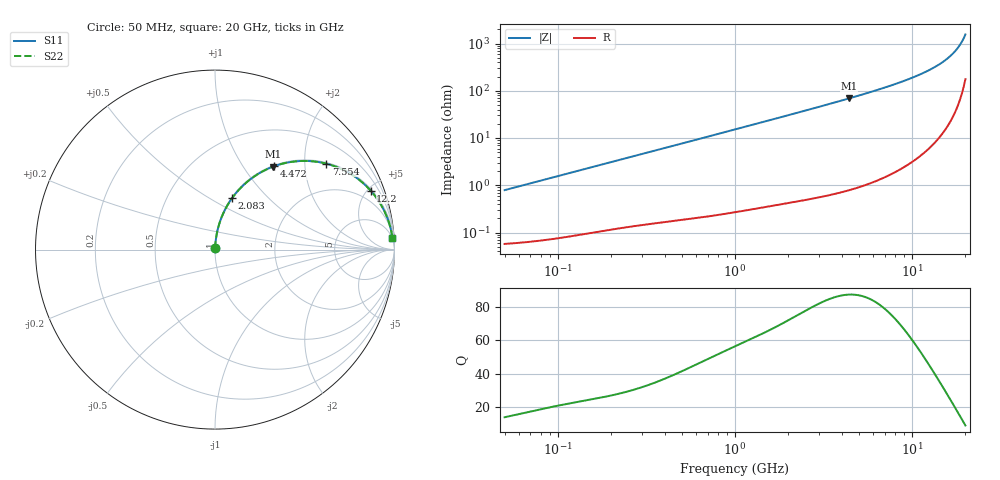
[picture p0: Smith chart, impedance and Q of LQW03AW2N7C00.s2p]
!Murata Part Number: LQW03AW2N7C00
!These Parameters are Measured in Series Mode Connection
!  o--[Z]--o
!Port1  Port2
!  o-------o
!Freq. Start=50[MHz] Stop=20[GHz], 401[Steps]
# Hz S RI R 50
!Freq.(Hz) S11(Real) S11(Imag) S21(Real) S21(Imag) S12(Real) S12(Imag) S22(Real) S22(Imag)
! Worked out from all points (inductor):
!   401 points, 50 MHz to 20 GHz, reference 50 ohm
!   read as one part in series: L = 2.51 nH near 51.52 MHz
!   highest Q = 87.6 at 4.406 GHz (marker M1), where L = 2.49 nH
!   S11 on the Smith chart (normalised r, x): 50 MHz: 1.00, +0.02; 2.083 GHz: 1.01, +0.63; 4.472 GHz: 1.02, +1.40; 7.554 GHz: 1.03, +2.57; 12.2 GHz: 1.11, +5.24; 20 GHz: 5, +31
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5e7  0.000637 0.00788  0.9994 -0.00788  0.9994 -0.00788  0.000637 0.00788
1.364002e8  0.00136 0.0212  0.9986 -0.0212  0.9986 -0.0212  0.00136 0.0212
3.721004e8  0.00483 0.0567  0.9952 -0.0567  0.9952 -0.0567  0.00483 0.0567
6.285508e8  0.0111 0.0946  0.9889 -0.0946  0.9889 -0.0946  0.0111 0.0946
1e9  0.0251 0.1478  0.9749 -0.1478  0.9749 -0.1478  0.0251 0.1478
1.498439e9  0.0523 0.215  0.9477 -0.215  0.9477 -0.215  0.0523 0.215
2.083303e9  0.0946 0.2859  0.9054 -0.2859  0.9054 -0.2859  0.0946 0.2859
2.728004e9  0.1514 0.3523  0.8486 -0.3523  0.8486 -0.3523  0.1514 0.3523
3.466789e9  0.2251 0.4118  0.7749 -0.4118  0.7749 -0.4118  0.2251 0.4118
4.405649e9  0.3242 0.4624  0.6758 -0.4624  0.6758 -0.4624  0.3242 0.4624
4.472136e9  0.3312 0.465  0.6688 -0.465  0.6688 -0.465  0.3312 0.465
5.856089e9  0.4725 0.4934  0.5275 -0.4934  0.5275 -0.4934  0.4725 0.4934
7.442007e9  0.6118 0.4809  0.3882 -0.4809  0.3882 -0.4809  0.6118 0.4809
7.554318e9  0.6205 0.4787  0.3795 -0.4787  0.3795 -0.4787  0.6205 0.4787
9.745021e9  0.7628 0.4174  0.2372 -0.4174  0.2372 -0.4174  0.7628 0.4174
1.220001e10  0.8676 0.3284  0.1324 -0.3284  0.1324 -0.3284  0.8676 0.3284
1.438523e10  0.9261 0.2476  0.0739 -0.2476  0.0739 -0.2476  0.9261 0.2476
1.646126e10  0.9608 0.1746  0.0392 -0.1746  0.0392 -0.1746  0.9608 0.1746
1.800918e10  0.977 0.1237  0.023 -0.1237  0.023 -0.1237  0.977 0.1237
1.855685e10  0.9811 0.1064  0.0189 -0.1064  0.0189 -0.1064  0.9811 0.1064
1.940974e10  0.9862 0.0803  0.0138 -0.0803  0.0138 -0.0803  0.9862 0.0803
2e10  0.9888 0.0628  0.0112 -0.0628  0.0112 -0.0628  0.9888 0.0628
